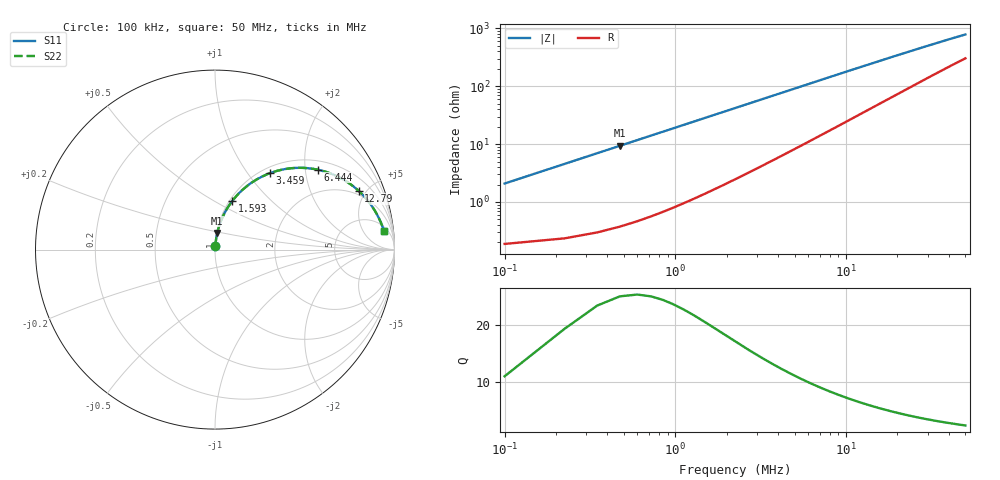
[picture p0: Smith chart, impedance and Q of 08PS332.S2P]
! Coilcraft 0805PS-332 Power Chip Inductor
! 5 February 2003
# MHZ S MA R 50
!Freq  MagS11  AngS11  MagS21  AngS21  MagS12  AngS12  MagS22  AngS22
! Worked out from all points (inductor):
!   403 points, 100 kHz to 50 MHz, reference 50 ohm
!   read as one part in series: L = 3.15 uH near 348.8 kHz
!   highest Q = 23.7 at 473.2 kHz (marker M1), where L = 3.15 uH
!   S11 on the Smith chart (normalised r, x): 100 kHz: 1.00, +0.04; 1.593 MHz: 1.03, +0.61; 3.459 MHz: 1.09, +1.28; 6.444 MHz: 1.24, +2.33; 12.79 MHz: 1.72, +4.46; 50 MHz: 7, +15
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0.1  0.02075 83.6  0.9979 -1.2  0.9979 -1.2  0.02075 83.6
0.2244  0.04533 84.5  0.9966 -2.6  0.9966 -2.6  0.04533 84.5
0.3488  0.0694 83.6  0.9946 -4.0  0.9946 -4.0  0.0694 83.6
0.4732  0.09306 82.4  0.992 -5.3  0.992 -5.3  0.09306 82.4
0.5976  0.1163 81.1  0.9886 -6.7  0.9886 -6.7  0.1163 81.1
0.722  0.1392 79.7  0.9847 -8.0  0.9847 -8.0  0.1392 79.7
0.9708  0.1837 77.0  0.9753 -10.6  0.9753 -10.6  0.1837 77.0
1.2196  0.2265 74.3  0.9638 -13.1  0.9638 -13.1  0.2265 74.3
1.5928  0.2872 70.5  0.9437 -16.7  0.9437 -16.7  0.2872 70.5
1.966  0.3435 66.8  0.9206 -20.1  0.9206 -20.1  0.3435 66.8
2.4636  0.4115 62.3  0.8867 -24.3  0.8867 -24.3  0.4115 62.3
3.4588  0.5244 54.3  0.8142 -31.5  0.8142 -31.5  0.5244 54.3
4.7028  0.6285 46.3  0.7255 -38.8  0.7255 -38.8  0.6285 46.3
6.4444  0.7248 37.9  0.6178 -46.1  0.6178 -46.1  0.7248 37.9
8.4348  0.7919 31.2  0.5214 -51.8  0.5214 -51.8  0.7919 31.2
10.4252  0.8335 26.3  0.4482 -55.6  0.4482 -55.6  0.8335 26.3
12.7888  0.865 22.2  0.3828 -58.6  0.3828 -58.6  0.865 22.2
16.7696  0.8955 17.5  0.3067 -61.6  0.3067 -61.6  0.8955 17.5
25.1044  0.924 12.1  0.2171 -63.6  0.2171 -63.6  0.924 12.1
33.4392  0.9364 9.3  0.1693 -63.4  0.1693 -63.4  0.9364 9.3
41.774  0.9431 7.5  0.1399 -62.3  0.1399 -62.3  0.9431 7.5
50  0.9473 6.4  0.1202 -60.9  0.1202 -60.9  0.9473 6.4
